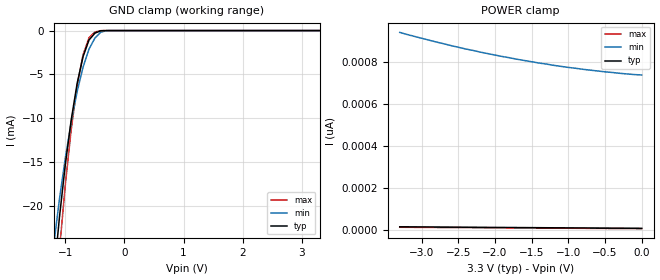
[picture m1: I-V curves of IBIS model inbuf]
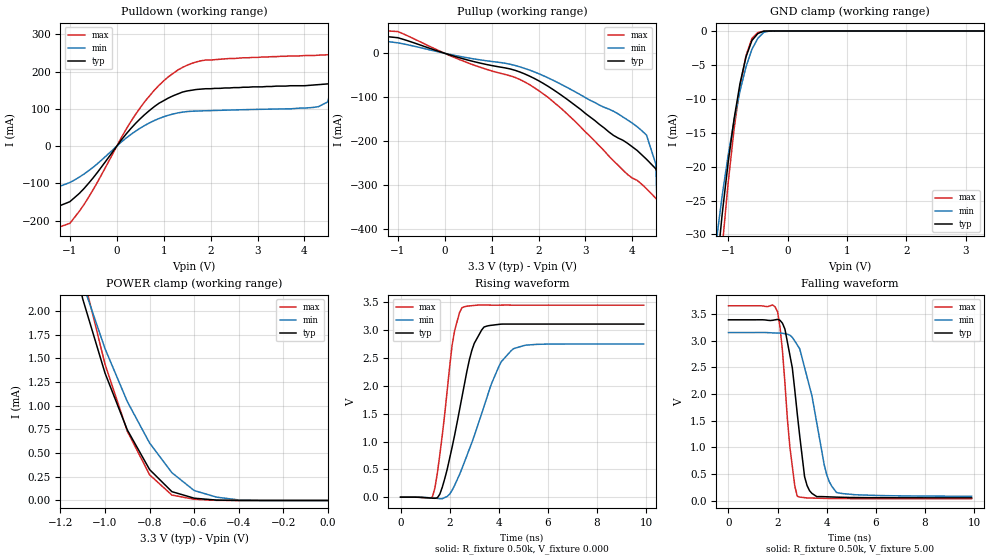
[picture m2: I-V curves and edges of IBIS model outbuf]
| IBIS file 43805p.ibs created by s2ibis2 version 1.0
| North Carolina State University Electronics Research Laboratory  1995
[IBIS ver]   2.1
[File name]   43805p.ibs
[File Rev]   0.1
[Date]   Wednesday, March 12, 1997
[Source]   IDT
[Notes]   1. Temp typ=25C, min=100C, max=0C 2. Ramp rates based on 500
   ohm load
[Copyright]   Copyright 1997, Integrated Device Technology, Inc.
[Disclaimer] Integrated Device Technology, Inc. ("IDT") hereby grants the
   user of this IBIS model a non-exclusive, nontransferable
   license to use this IBIS model under the following terms.
   The user is granted this license only to use the IBIS model
   and is not granted rights to sell, copy (except as needed to
   run the IBIS model), rent, lease or sub-license the IBIS model
   in whole or in part, or in modified form to anyone.
   The User may modify the IBIS model to suit its specific
   applications, but rights to derivative works and such
   modifications shall belong to IDT.
   This IBIS model is provided on an "AS IS" basis and IDT
   makes absolutely no warranty with respect to the information
   contained herein. IDT DISCLAIMS AND CUSTOMER WAIVES ALL
   WARRANTIES, EXPRESS AND IMPLIED, INCLUDING WARRANTIES OF
   MERCHANTABILITY AND FITNESS FOR A PARTICULAR PURPOSE. THE
   ENTIRE RISK AS TO QUALITY AND PERFORMANCE IS WITH THE
   USER ACCORDINGLY, IN NO EVENT SHALL IDT BE LIABLE
   FOR ANY DIRECT OR INDIRECT DAMAGES, WHETHER IN CONTRACT OR
   TORT, INCLUDING ANY LOST PROFITS OR OTHER INCIDENTAL,
   CONSEQUENTIAL, EXEMPLARY, OR PUNITIVE DAMAGES ARISING OUT OF
   THE USE OR APPLICATION OF THE IBIS model.  Further, IDT
   reserves the right to make changes without notice to any
   product herein to improve reliability, function, or design.
   IDT does not convey any license under patent rights or
   any other intellectual property rights, including those of
   third parties. IDT is not obligated to provide maintenance
   or support for the licensed IBIS model.
|   Component IDT49FCT3805/A
[Component]   IDT49FCT3805/A
[Manufacturer]   Integrated Device Technology Inc.
[Package]
| Following package parameters are for D20-1(CDIP), P20-1(DPIP) packages
|[Package]
|| variable   typ   min   max
|R_pkg   40.00m   30.00m   50.00m
|L_pkg   7.00nH   4.00nH   10.00nH
|C_pkg   0.60pF   0.50pF   0.70pF
| Following package parameters are for SO20-6(EIAJ), SO20-2(SOIC) packages
|[Package]
|| variable   typ   min   max
|R_pkg   25.00m   20.00m   30.00m
|L_pkg   3.50nH   2.10nH   6.50nH
|C_pkg   0.40pF   0.35pF   0.60pF
| Following package parameters are for SO20-8(QSOP), SO20-7(SSOP) packages
| variable   typ   min   max
R_pkg   20.00m   15.00m   25.00m
L_pkg   3.00nH   2.00nH   4.00nH
C_pkg   0.30pF   0.26pF   0.34pF
[Pin]  signal_name   model_name   R_pin   L_pin   C_pin
1   VCCA   POWER
2   OA1   outbuf
3   OA2   outbuf
4   OA3   outbuf
5   GNDA   GND
6   OA4   outbuf
7   OA5   outbuf
8   GNDQ   GND
9   OEAB   inbuf
10   INA   inbuf
11   INB   inbuf
12   OEBB   inbuf
13   MON   outbuf
14   OB5   outbuf
15   OB4   outbuf
16   GNDB   GND
17   OB3   outbuf
18   OB2   outbuf
19   OB1   outbuf
20   VCCB   POWER
| Models and submodels in the file (2): inbuf (Input), outbuf (3-state)
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| in   IN1   dummy_model
| oe   OE1   dummy_model
|   Model inbuf
[Model]   inbuf
Model_type   Input
Vinl =  0.800V
Vinh =  2.000V
C_comp   3.00pF   NA   NA
[Temperature Range]   25.00   100.00   0.000
[Voltage Range]   3.30V   3.00V   3.60V
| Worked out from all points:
|   GND clamp passes 1 mA (typ) near -0.59 V on its own axis
[GND_clamp]
| voltage   I(typ)   I(min)   I(max)
-3.3V     -32.08A    -29.15A    -33.09A
-1.2V     -28.45mA   -24.7mA    -34.05mA
-1.1V     -21.32mA   -19.24mA   -25.12mA
-1V       -15.28mA   -14.53mA   -17.56mA
-900mV    -10.16mA   -10.42mA   -11.24mA
-800mV    -6.017mA   -6.948mA   -6.255mA
-700mV    -2.962mA   -4.157mA   -2.751mA
-600mV    -1.078mA   -2.117mA   -816uA
-500mV    -294uA     -855uA     -169uA
-400mV    -19.55uA   -178uA     -9.254uA
-300mV    -240nA     -7.217uA   -67.1nA
3.3V      8.95pA     748pA      6.811pA
[POWER_clamp]
| voltage   I(typ)   I(min)   I(max)
-3.3V     16.3pA     943pA      14.06pA
-3.2V     16.07pA    933pA      13.89pA
-2.8V     15.13pA    897pA      13.07pA
-2.4V     14.22pA    864pA      12.26pA
-2.2V     13.77pA    849pA      11.84pA
-1.7V     12.65pA    815pA      10.83pA
-1.2V     11.54pA    786pA      9.836pA
-800mV    10.66pA    767pA      9.029pA
-300mV    9.58pA     748pA      8.014pA
-100mV    9.152pA    742pA      7.608pA
0V        8.945pA    740pA      7.396pA
|   Model outbuf
[Model]   outbuf
Model_type   3-state
Polarity   Non-Inverting
Enable   Active-High
Vinl =  0.800V
Vinh =  2.000V
C_comp   3.00pF   NA   NA
[Temperature Range]   25.00   100.00   0.000
[Voltage Range]   3.30V   3.00V   3.60V
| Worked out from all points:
|   slope of the pulldown table from 0 to 0.495 V, typ, clamps not added: 6.79 ohm
|   slope of the pullup table from 0 to 0.495 V, typ, clamps not added: 32.1 ohm
|   GND clamp passes 1 mA (typ) near -0.56 V on its own axis
|   POWER clamp passes 1 mA (typ) near -0.94 V on its own axis
|   rising waveform, R_fixture 0.50k, V_fixture 0.000: 20-80 % time 854ps typ, 1.33ns min, 534ps max; typ from 0 V to 3.11 V
|   falling waveform, R_fixture 0.50k, V_fixture 5.00: 20-80 % time 526ps typ, 814ps min, 396ps max; typ from 3.39 V to 0.057 V
[Pulldown]
| voltage   I(typ)   I(min)   I(max)
-3.3V     -10mA      -10mA      -10mA
-1.9V     -39mA      -45mA      -46mA
-1.5V     -174mA     -121mA     -229mA
-1V       -149mA     -97.58mA   -207mA
500mV     73.5mA     48.28mA    103mA
1.4V      145mA      91.23mA    211mA
4.3V      165mA      106mA      244mA
4.5V      167mA      119mA      245mA
4.7V      175mA      243mA      247mA
4.9V      293mA      575mA      252mA
5.3V      1.108A     1.487A     599mA
6.6V      4.493A     4.866A     3.897A
[Pullup]
| voltage   I(typ)   I(min)   I(max)
-3.3V     2mA        2mA        2mA
-1.9V     9.1mA      10.2mA     10.7mA
-1.7V     18.3mA     20.4mA     21mA
-1.5V     40.75mA    30.62mA    52.61mA
-1V       35.47mA    23.79mA    49.47mA
1.9V      -56.69mA   -41.91mA   -77.53mA
3.7V      -193mA     -138mA     -255mA
4.3V      -241mA     -186mA     -308mA
4.5V      -263mA     -252mA     -330mA
4.7V      -308mA     -954mA     -356mA
4.9V      -962mA     -3.632A    -389mA
6.6V      -40.31A    -44.16A    -33.99A
[GND_clamp]
| voltage   I(typ)   I(min)   I(max)
-3.3V     -40.25A    -36.52A    -41.58A
-1.2V     -35.85mA   -31.05mA   -43.02mA
-1.1V     -26.94mA   -24.22mA   -31.86mA
-1V       -19.37mA   -18.32mA   -22.39mA
-900mV    -12.93mA   -13.18mA   -14.44mA
-800mV    -7.703mA   -8.803mA   -8.116mA
-700mV    -3.816mA   -5.277mA   -3.621mA
-600mV    -1.39mA    -2.686mA   -1.083mA
-500mV    -367uA     -1.072mA   -228uA
-400mV    -19.15uA   -190uA     -8.456uA
-300mV    -246nA     -7.762uA   -65.09nA
3.3V      134pA      576nA      125pA
[POWER_clamp]
| voltage   I(typ)   I(min)   I(max)
-3.3V     4.316A     3.959A     4.439A
-1.1V     2.125mA    2.288mA    2.388mA
-1V       1.343mA    1.601mA    1.437mA
-900mV    744uA      1.043mA    730uA
-800mV    326uA      606uA      271uA
-700mV    93.08uA    293uA      57.1uA
-600mV    24.29uA    105uA      12.74uA
-500mV    4.099uA    35.49uA    1.42uA
-400mV    216nA      5.651uA    54.69nA
0V        134pA      675pA      144pA
[Ramp]
| variable   typ   min   max
dV/dt_r   1.87/0.85n   1.65/1.33n   2.07/0.53n
dV/dt_f   1.96/0.50n   1.77/0.81n   2.14/0.38n
R_load = 0.50k
[Rising Waveform]
R_fixture = 0.50k
V_fixture = 0.000
| time   V(typ)   V(min)   V(max)
0s        0V         0V         0V
1.3ns     -18.32mV   -14.06mV   5.698mV
1.6ns     53.35mV    -27.96mV   762mV
2.1ns     897mV      123mV      2.729V
2.5ns     1.795V     511mV      3.405V
2.9ns     2.632V     976mV      3.441V
3.3ns     3.002V     1.498V     3.454V
4ns       3.105V     2.345V     3.451V
4.6ns     3.111V     2.669V     3.451V
9.9ns     3.111V     2.753V     3.451V
[Falling Waveform]
R_fixture = 0.50k
V_fixture = 5.00
| time   V(typ)   V(min)   V(max)
0s        3.392V     3.153V     3.655V
2ns       3.4V       3.143V     3.544V
2.3ns     3.217V     3.131V     2.21V
2.5ns     2.734V     3.104V     1.016V
2.8ns     1.641V     2.923V     87.27mV
3.1ns     453mV      2.498V     60.17mV
3.2ns     289mV      2.321V     54.54mV
4ns       76.58mV    493mV      45.65mV
4.4ns     69.81mV    157mV      43.28mV
9.9ns     56.85mV    86.78mV    40.88mV
